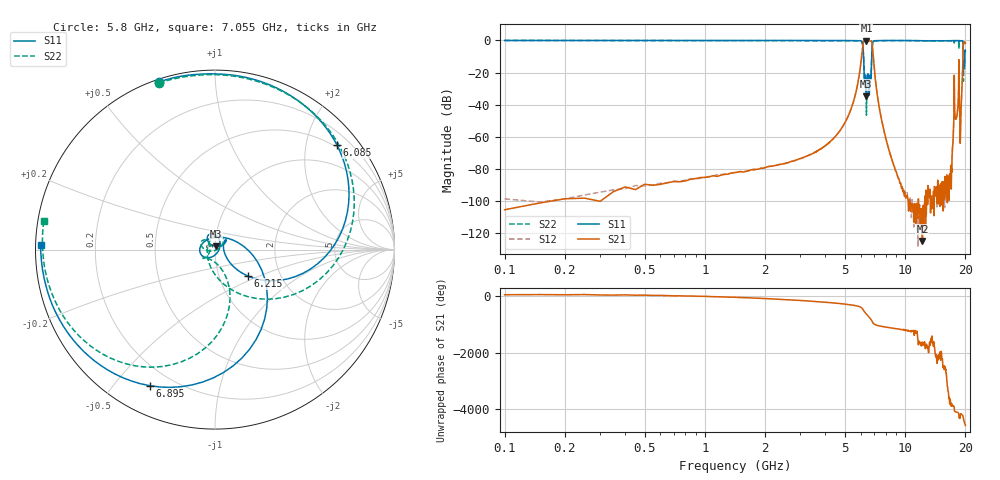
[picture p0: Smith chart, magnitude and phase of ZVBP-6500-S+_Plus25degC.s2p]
! Mini-Circuits
! S2P DATA File Format
! Type: BAND PASS FILTER
! Model: ZVBP-6500-S+
! All S Parameters are in dB deg format
! TEST CONDITIONS: INPUT POWER = 0 dBm @ Temperature = +25deg C
# MHZ S DB R 50
!Frequency  S11 dB  S11 DEG  S21 dB  S21 DEG  S12 dB  S12 DEG  S22 dB  S22 DEG
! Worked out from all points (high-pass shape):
!   1299 points, 100 MHz to 20 GHz, reference 50 ohm
!   highest |S21| = -0.26 dB at 6.41 GHz (marker M1); lowest = -124.8 dB at 12.2 GHz (marker M2)
!   |S21| within 3 dB of the highest: 6.148 GHz to 6.857 GHz (708.6 MHz wide, 10.9 % of centre); 19.52 GHz to end of sweep
!   lowest |S11| = -34.7 dB at 6.405 GHz (marker M3), VSWR 1.04, Z = 50.5 + j1.78 ohm
!   |S11| at or under -10 dB: 6.202 GHz to 6.809 GHz (607.1 MHz wide, 9.33 % of centre); 19.52179 GHz to 19.5888 GHz (67 MHz wide, 0.343 % of centre); 19.71 GHz to 19.84 GHz (129.2 MHz wide, 0.653 % of centre)
!   |S22| runs from -46.6 to 0.0 dB; largest |S21 - S12| = 0.00077
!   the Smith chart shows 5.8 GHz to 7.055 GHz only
!   S11 on the Smith chart (normalised r, x): 5.8 GHz: 0.01, +0.72; 6.085 GHz: 0.45, +2.64; 6.215 GHz: 1.37, -0.43; 6.895 GHz: 0.12, -0.62; 7.055 GHz: 0.01, +0.01
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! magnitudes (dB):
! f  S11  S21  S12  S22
! 100 MHz  0.0  -105.3  -98.6  0.0
! 250 MHz  -0.1  -98.1  -96.2  -0.1
! 600 MHz  -0.1  -89.6  -88.9  -0.1
! 1.45 GHz  -0.1  -82.0  -82.0  -0.1
! 3.45 GHz  -0.1  -70.4  -70.3  -0.1
! 4.835 GHz  -0.1  -54.3  -54.4  -0.2
! 5.8 GHz  -0.1  -27.0  -27.0  -0.2
! 6.085 GHz  -1.0  -8.3  -8.3  -1.0
! 6.215 GHz  -12.6  -0.6  -0.6  -12.8
! 6.405 GHz  -34.7  -0.3  -0.3  -41.9
! 6.41 GHz  -34.6  -0.3  -0.3  -46.6
! 6.505 GHz  -20.9  -0.3  -0.3  -21.2
! 6.63 GHz  -32.5  -0.3  -0.3  -30.5
! 6.895 GHz  -1.5  -6.6  -6.6  -1.5
! 7.055 GHz  -0.2  -20.9  -20.9  -0.3
! 8.275 GHz  -0.1  -67.4  -67.5  -0.1
! 12.2 GHz  -0.2  -124.8  -108.7  -0.3
! 16.8 GHz  -0.2  -87.4  -87.9  -0.3
! 17.7 GHz  -0.1  -45.0  -45.0  -0.3
! 19 GHz  -0.2  -44.8  -44.8  -0.3
! 19.55 GHz  -18.0  -1.2  -1.2  -25.4
! 20 GHz  -6.8  -1.7  -1.7  -7.1
